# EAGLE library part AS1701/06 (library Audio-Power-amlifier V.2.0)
The AS1701 and AS1706 are 1.6W bridged audio power amplifiers that provide excellent circuit reliability, providing a very low-cost solution by eliminating external components when used with 2.7 to 5.5Vpowered circuits.
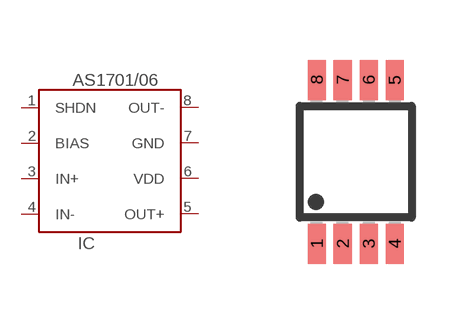
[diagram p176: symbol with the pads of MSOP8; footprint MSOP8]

Designator prefix IC

## AS1701/06  [MSOP8]
1  SHDN
2  BIAS
3  IN+  in
4  IN-  in
5  OUT+  out
6  VDD  pwr
7  GND  pwr
8  OUT-  out

## Footprint MSOP8 (pad centres in mm)
Micro Small Outline Package Grid .65mm
smd 0.45 x 1: 1 -0.975,-2.05; 2 -0.325,-2.05; 3 0.325,-2.05; 4 0.975,-2.05; 5 0.975,2.05; 6 0.325,2.05; 7 -0.325,2.05; 8 -0.975,2.05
